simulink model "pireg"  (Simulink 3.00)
settings: Solver=ode45  StartTime=0.0  StopTime=20  MaxStep=0.1  RelTol=1e-3  AbsTol=1e-3
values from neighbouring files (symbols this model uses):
  omega = 1    [eksper.m]    (also in eksper_sim_step.m)
undefined symbols (not defined in the file or in its folder): sfuny, zeta

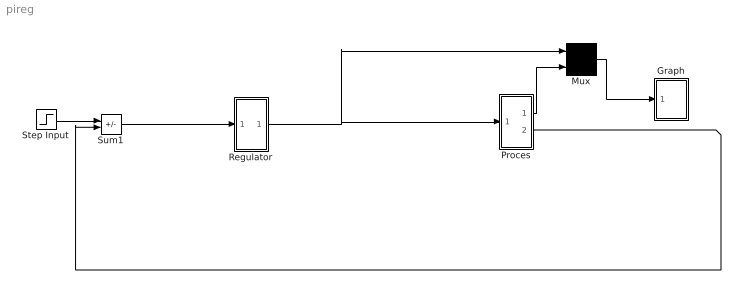
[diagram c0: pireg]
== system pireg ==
  Graph : Subsystem  LoadFcn=sfuny([],[],[],'LoadBlock')  StartFcn=sfuny([],[],[],'Start')  StopFcn=sfuny([],[],[],'Stop')  mask(Graph scope.){}
      mask help: Graph scope using MATLAB graph window. Enter plotting ranges and line type.
      mask init:
      | color = @4; ax = [0, @1, @2, @3]; dt = -1;
  Mux : Mux  Inputs=3
  Proces : Subsystem
  Regulator : Subsystem  mask(Pi reg){}
      mask help: Parametra:
      mask init:
      | kp=@1;ti=@2;
  Step Input : Step  Time=1  Before=0  After=1  SampleTime=-1
  Sum1 : Sum  Inputs=+-  SaturateOnIntegerOverflow=on
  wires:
  Step Input/1 -> Sum1/1
  Proces/2(out_2) -> Sum1/2
  Sum1/1 -> Regulator/1(in_1)
  Proces/1(out_1) -> Mux/3
  Regulator/1(out_1) -> Proces/1(in_1), Mux/1
  Mux/1 -> Graph/1(x)

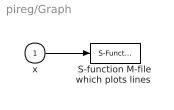
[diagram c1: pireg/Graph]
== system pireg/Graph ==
  x : Inport  Port=1  PortWidth=-1  SampleTime=-1  DataType=auto
  "S-function M-file which plots lines " : S-Function  FunctionName=sfuny  Parameters=ax, color,dt  PortCounts=[]  SFunctionModules=''
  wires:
  x/1 -> "S-function M-file which plots lines "/1

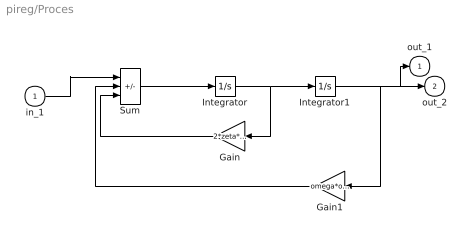
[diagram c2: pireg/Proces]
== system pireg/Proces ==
  in_1 : Inport  Port=1  PortWidth=-1  SampleTime=-1  DataType=auto
  Gain : Gain  Orientation=left  Gain=2*zeta*omega  SaturateOnIntegerOverflow=on
  Gain1 : Gain  Orientation=left  Gain=omega*omega  SaturateOnIntegerOverflow=on
  Integrator : Integrator  ExternalReset=none  InitialConditionSource=internal  InitialCondition=0  LimitOutput=off  UpperSaturationLimit=inf  LowerSaturationLimit=-inf  ShowSaturationPort=off  ShowStatePort=off  AbsoluteTolerance=auto
  Integrator1 : Integrator  ExternalReset=none  InitialConditionSource=internal  InitialCondition=0  LimitOutput=off  UpperSaturationLimit=inf  LowerSaturationLimit=-inf  ShowSaturationPort=off  ShowStatePort=off  AbsoluteTolerance=auto
  Sum : Sum  Inputs=+--  SaturateOnIntegerOverflow=on
  out_1 : Outport  Port=1
  out_2 : Outport  Port=2
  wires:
  Gain/1 -> Sum/3
  Integrator/1 -> Integrator1/1, Gain/1
  Gain1/1 -> Sum/2
  Sum/1 -> Integrator/1
  in_1/1 -> Sum/1
  Integrator1/1 -> Gain1/1, out_1/1, out_2/1

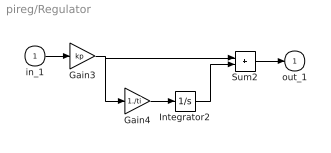
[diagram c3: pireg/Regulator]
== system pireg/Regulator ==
  in_1 : Inport  Port=1  PortWidth=-1  SampleTime=-1  DataType=auto
  Gain3 : Gain  Gain=kp  SaturateOnIntegerOverflow=on
  Gain4 : Gain  Gain=1./ti  SaturateOnIntegerOverflow=on
  Integrator2 : Integrator  ExternalReset=none  InitialConditionSource=internal  InitialCondition=0  LimitOutput=off  UpperSaturationLimit=inf  LowerSaturationLimit=-inf  ShowSaturationPort=off  ShowStatePort=off  AbsoluteTolerance=auto
  Sum2 : Sum  Inputs=++  SaturateOnIntegerOverflow=on
  out_1 : Outport  Port=1
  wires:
  Integrator2/1 -> Sum2/2
  Gain4/1 -> Integrator2/1
  Gain3/1 -> Sum2/1, Gain4/1
  in_1/1 -> Gain3/1
  Sum2/1 -> out_1/1
